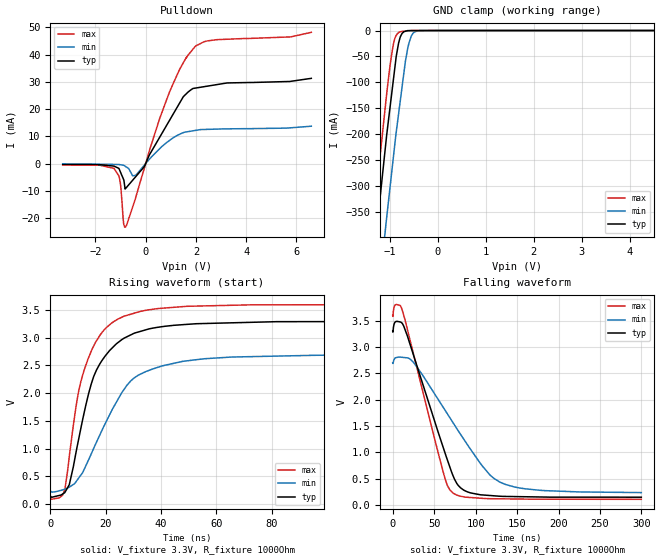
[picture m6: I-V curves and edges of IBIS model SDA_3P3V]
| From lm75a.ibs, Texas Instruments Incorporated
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|   Model SDA_3P3V
[Model]   SDA_3P3V
Model_type   I/O_open_drain
Polarity   Non-Inverting
Enable   Active-Low
Vinl = .99
Vinh = 2.31
Vmeas = 1.65
Vref = 3.3
Cref = 15pF
Rref = 1000
|   typ   min   max
|   (nom PVT)   (fast PVT)   (slow PVT)
C_comp   0.589p   0.536p   0.668p
|C_comp (ON state)   0.589p   0.536p   0.668p
|C_comp (OFF state)   0.700p   0.696p   0.721p
| Where   nom PVT is  Nominal Process, 3.3V, 27C
|   Fast PVT is Strong Process, 3.6V, -40C
|   Slow PVT is Weak Process, 2.7V, 150C
[Model spec]
|subparameter
Vinl   0.99   0.81   1.08
Vinh   2.31   1.89   2.52
[Voltage Range]   3.3   2.7   3.6
[Temperature Range]   27   150   -40
[Pullup Reference]   3.3   2.7   3.6
[Pulldown Reference]   0   0   0
[Power Clamp Reference]   3.3   2.7   3.6
[GND Clamp Reference]   0   0   0
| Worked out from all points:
|   slope of the pulldown table from 0 to 0.495 V, typ, clamps not added: 57.1 ohm
|   GND clamp passes 1 mA (typ) near -0.66 V on its own axis
|   falling waveform, V_fixture 3.3V, R_fixture 1000Ohm: 20-80 % time 39ns typ, 62.1ns min, 33.3ns max; typ from 3.3 V to 0.148 V
|   rising waveform, V_fixture 3.3V, R_fixture 1000Ohm: 20-80 % time 11.1ns typ, 15.6ns min, 9.43ns max; typ from 0.145 V to 3.3 V
[Pulldown]
|   Voltage   I(typ)   I(min)   I(max)
-3.3V     -367.1uA   -119uA     -531.5uA
-1.259V   -962.4uA   -335.7uA   -1.789mA
-1.012V   -2.938mA   -446.3uA   -6.854mA
-875.5mV  -5.904mA   -646.5uA   -22.01mA
-804.1mV  -9.215mA   -1.066mA   -23.35mA
-405.2mV  -4.934mA   -4.391mA   -12.78mA
-51.84mV  -1.142mA   -574.8uA   -1.723mA
951.9mV   15.88mA    8.496mA    26.33mA
1.496V    24.49mA    11.32mA    36.94mA
1.958V    27.65mA    12.11mA    42.83mA
2.818V    28.93mA    12.63mA    45.44mA
6.59V     31.25mA    13.69mA    48.14mA
[GND Clamp]
|   Voltage   I(typ)   I(min)   I(max)
-3.3V     -2.268A    -2.367A    -2.221A
-1.457V   -550.3mA   -703.8mA   -472.2mA
-1.271V   -381.5mA   -538.6mA   -301.2mA
-1.073V   -207.6mA   -366.2mA   -128.1mA
-937.3mV  -103mA     -253mA     -31.39mA
-867.1mV  -49.49mA   -195.5mA   -9.285mA
-804.1mV  -19.28mA   -150.5mA   -3.089mA
-677.4mV  -1.454mA   -59.94mA   -1.083mA
-603.2mV  -169.2uA   -24.51mA   -442.1uA
-516.6mV  -142.6uA   -5.083mA   0A
-405.2mV  -108.4uA   -318.6uA   0A
6.59V     0A         0A         0A
[Ramp]
R_load = 1000
|   typ   min   max
dV/dt_r   1.8927/1.10886e-08   1.48059/1.56123e-08   2.09539/9.43153e-09
dV/dt_f   1.89092/3.88089e-08   1.47851/6.19559e-08   2.09534/3.32397e-08
[Falling Waveform]
V_fixture = 3.3V
V_fixture_min = 2.7V
V_fixture_max = 3.6V
R_fixture = 1000Ohm
C_fixture = 0F
|   Time   V(typ)   V(min)   V(max)
0s        3.3V       2.7V       3.6V
3.245ns   3.48V      2.797V     3.805V
11.02ns   3.459V     2.807V     3.728V
25.82ns   2.812V     2.696V     2.823V
62.02ns   1.041V     1.829V     561.7mV
73.01ns   548.2mV    1.558V     223.5mV
89.68ns   252mV      1.157V     147mV
117.3ns   180.5mV    570.9mV    119.9mV
136.5ns   162.8mV    387.9mV    116.4mV
299.9ns   148.5mV    235.8mV    107.8mV
[Rising Waveform]
V_fixture = 3.3V
V_fixture_min = 2.7V
V_fixture_max = 3.6V
R_fixture = 1000Ohm
C_fixture = 0F
|   Time   V(typ)   V(min)   V(max)
0s        145.5mV    232.3mV    107.7mV
5.266ns   206.1mV    266.8mV    260.3mV
6.863ns   347.1mV    303mV      852.8mV
10.22ns   1.161V     463.5mV    2.027V
15.12ns   2.214V     940.1mV    2.796V
21.4ns    2.768V     1.607V     3.233V
27.68ns   3.018V     2.141V     3.404V
32.59ns   3.115V     2.343V     3.477V
65.51ns   3.269V     2.651V     3.586V
299.9ns   3.3V       2.7V       3.6V
